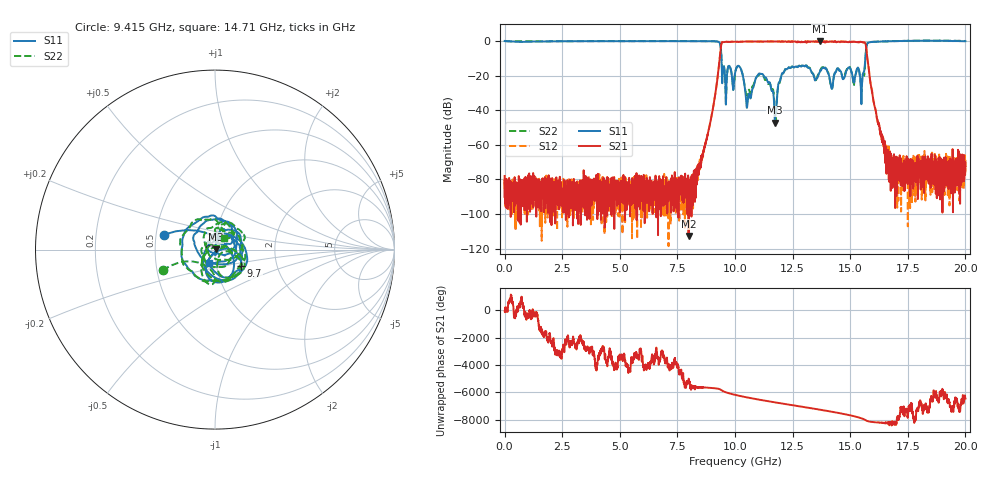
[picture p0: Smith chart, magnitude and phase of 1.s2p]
!Keysight Technologies,N5232A,MY52221221,A.10.65.11
!Date: Tuesday, September 24, 2024 11:59:07
!Correction: S11(Full 2 Port(1,4))
!S41(Full 2 Port(1,4))
!S14(Full 2 Port(1,4))
!S44(Full 2 Port(1,4))
!S2P File: Measurements: S11, S41, S14, S44:
# Hz S  RI  R 50
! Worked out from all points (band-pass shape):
!   4001 points, 300 kHz to 20 GHz, reference 50 ohm
!   highest |S21| = -0.06 dB at 13.69 GHz (marker M1); lowest = -112.7 dB at 7.985 GHz (marker M2)
!   |S21| within 3 dB of the highest: 9.39 GHz to 15.69 GHz (6.296 GHz wide, 50.2 % of centre)
!   lowest |S11| = -47.3 dB at 11.73 GHz (marker M3), VSWR 1.01, Z = 50.4 + j0.144 ohm
!   |S11| at or under -10 dB: 9.413 GHz to 15.65 GHz (6.24 GHz wide, 49.8 % of centre)
!   |S22| runs from -45.9 to 0.3 dB; largest |S21 - S12| = 0.082
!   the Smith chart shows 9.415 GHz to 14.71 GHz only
!   S11 on the Smith chart (normalised r, x): 9.415 GHz: 0.55, +0.10; 9.7 GHz: 1.31, -0.25; 14.71 GHz: 0.93, -0.14
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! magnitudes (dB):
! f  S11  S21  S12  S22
! 300 kHz  0.0  -78.0  -79.5  0.0
! 3.335 GHz  -0.1  -82.3  -83.1  -0.1
! 6.67 GHz  -0.1  -90.6  -93.4  -0.1
! 7.985 GHz  -0.1  -112.7  -80.2  0.0
! 8.7 GHz  -0.2  -59.2  -60.6  -0.1
! 9.275 GHz  -0.4  -17.5  -17.6  -0.4
! 9.415 GHz  -10.5  -1.3  -1.3  -10.1
! 9.7 GHz  -15.3  -0.5  -0.6  -15.0
! 10 GHz  -18.6  -0.4  -0.4  -19.1
! 10.22 GHz  -15.2  -0.5  -0.4  -15.1
! 10.58 GHz  -31.4  -0.3  -0.3  -28.9
! 11.18 GHz  -19.0  -0.3  -0.4  -20.3
! 11.73 GHz  -47.3  -0.2  -0.3  -43.4
! 12.24 GHz  -16.4  -0.5  -0.3  -16.5
! 13.34 GHz  -18.3  -0.3  -0.1  -18.1
! 13.69 GHz  -17.7  -0.1  -0.6  -17.7
! 14.71 GHz  -21.8  -0.4  -0.5  -21.9
! 15.51 GHz  -25.5  -0.6  -0.6  -24.1
! 15.63 GHz  -15.4  -0.9  -0.9  -17.7
! 15.81 GHz  -0.8  -16.5  -15.5  -0.8
! 16.67 GHz  -0.2  -69.2  -64.0  -0.1
! 20 GHz  -0.1  -72.3  -75.5  0.0
